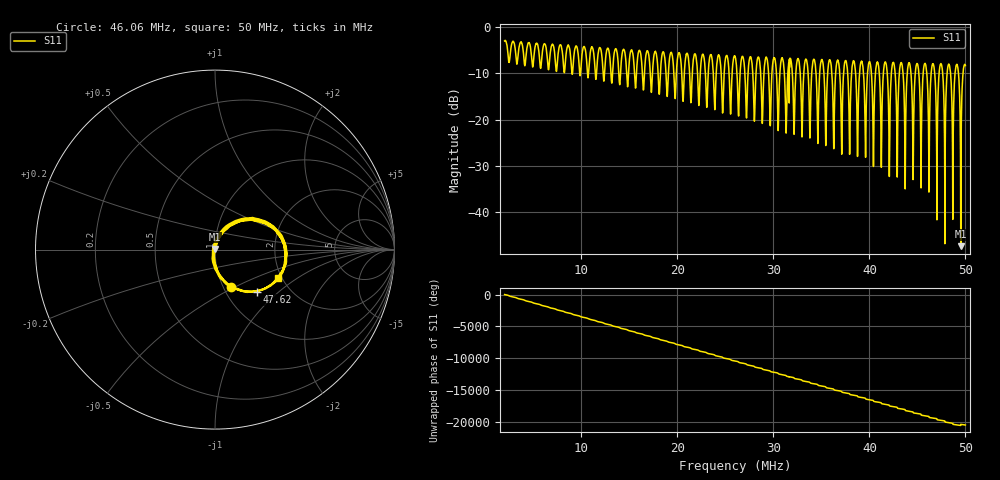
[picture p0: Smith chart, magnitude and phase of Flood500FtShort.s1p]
! ListType=Lin
!!500FtFloodedShort
# MHz S RI R 50
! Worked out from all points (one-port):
!   4096 points, 2 MHz to 50 MHz, reference 50 ohm
!   lowest |S11| = -47.4 dB at 49.52 MHz (marker M1), VSWR 1.01, Z = 50 + j0.426 ohm
!   |S11| at or under -10 dB: 46.81 MHz to 47.26 MHz (453.5 kHz wide, 0.964 % of centre); 47.64 MHz to 48.09 MHz (456.2 kHz wide, 0.953 % of centre); 49.28 MHz to 49.75 MHz (467.5 kHz wide, 0.944 % of centre)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
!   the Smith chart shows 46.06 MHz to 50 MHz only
!   S11 on the Smith chart (normalised r, x): 46.06 MHz: 1.08, -0.48; 47.62 MHz: 1.38, -0.73; 50 MHz: 1.90, -0.71
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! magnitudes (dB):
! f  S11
! 2 MHz  -3.0
! 8.001 MHz  -5.2
! 14 MHz  -12.2
! 20 MHz  -6.8
! 26.01 MHz  -6.4
! 32.01 MHz  -11.4
! 36.3 MHz  -26.3
! 36.7 MHz  -7.2
! 37.12 MHz  -27.5
! 37.53 MHz  -7.2
! 38.01 MHz  -18.0
! 38.35 MHz  -7.3
! 38.76 MHz  -28.0
! 39.17 MHz  -7.4
! 39.59 MHz  -28.1
! 40 MHz  -7.5
! 40.41 MHz  -28.2
! 40.82 MHz  -7.5
! 41.23 MHz  -29.2
! 41.64 MHz  -7.5
! 42.06 MHz  -30.9
! 44.01 MHz  -8.6
! 46.06 MHz  -12.9
! 47.62 MHz  -9.6
! 48.71 MHz  -29.8
! 49.12 MHz  -8.1
! 49.52 MHz  -47.4
! 50 MHz  -8.3
